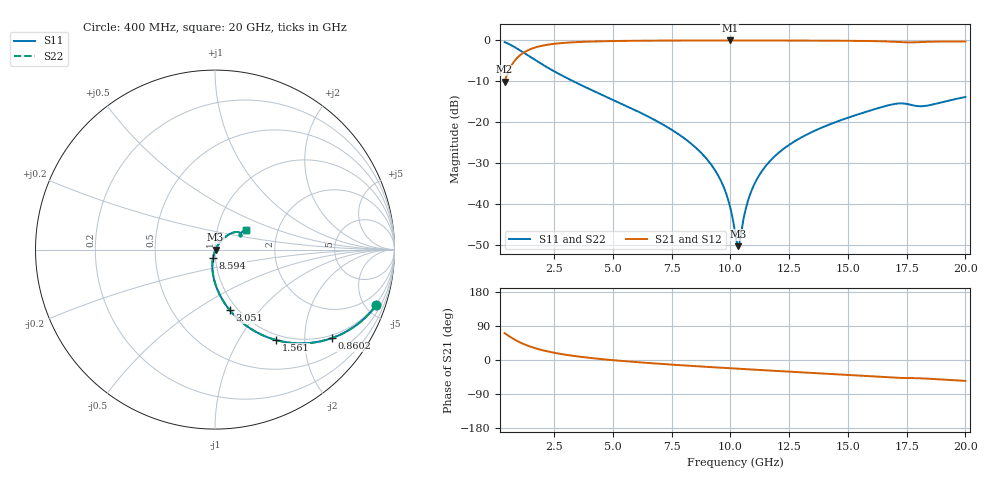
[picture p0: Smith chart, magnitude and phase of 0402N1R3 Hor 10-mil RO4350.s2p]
# GHz S MA R 50
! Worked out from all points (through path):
!   1960 points, 400 MHz to 20 GHz, reference 50 ohm
!   highest |S21| = -0.03 dB at 9.975 GHz (marker M1); lowest = -10.1 dB at 400 MHz (marker M2)
!   group delay of S21, straight-line fit = 12.9 ps
!   lowest |S11| = -50.3 dB at 10.34 GHz (marker M3), VSWR 1.01, Z = 50.3 - j0.116 ohm
!   |S11| at or under -10 dB: 3.318 GHz to end of sweep
!   |S22| runs from -50.3 to -0.4 dB; largest |S21 - S12| = 0
!   S11 on the Smith chart (normalised r, x): 400 MHz: 0.91, -5.82; 860.2 MHz: 0.91, -2.69; 1.561 GHz: 0.91, -1.46; 3.051 GHz: 0.92, -0.70; 8.594 GHz: 0.97, -0.09; 20 GHz: 1.38, +0.31
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0.4  0.9502 -19.0  0.3115 70.9  0.3115 70.9  0.9502 -19.0
0.8602348  0.8157 -37.2  0.5779 52.7  0.5779 52.7  0.8157 -37.2
1.560592  0.6081 -56.0  0.7928 33.9  0.7928 33.9  0.6081 -56.0
2.210924  0.4677 -66.9  0.8826 22.9  0.8826 22.9  0.4677 -66.9
3.051353  0.3456 -76.4  0.9367 13.4  0.9367 13.4  0.3456 -76.4
3.671669  0.2822 -81.5  0.9575 8.1  0.9575 8.1  0.2822 -81.5
6.943338  0.1005 -98.4  0.9922 -9.8  0.9922 -9.8  0.1005 -98.4
8.594181  0.04703 -103.2  0.9958 -16.5  0.9958 -16.5  0.04703 -103.2
9.444615  0.02335 -102.7  0.9964 -19.8  0.9964 -19.8  0.02335 -102.7
9.744768  0.01546 -99.9  0.9965 -20.9  0.9965 -20.9  0.01546 -99.9
9.974885  0.009648 -93.7  0.9965 -21.7  0.9965 -21.7  0.009648 -93.7
10.205  0.004449 -69.6  0.9965 -22.6  0.9965 -22.6  0.004449 -69.6
10.33507  0.003059 -22.1  0.9965 -23.0  0.9965 -23.0  0.003059 -22.1
10.4051  0.003573 7.4  0.9965 -23.3  0.9965 -23.3  0.003573 7.4
10.61521  0.007754 42.2  0.9964 -24.1  0.9964 -24.1  0.007754 42.2
10.7853  0.01176 49.8  0.9963 -24.7  0.9963 -24.7  0.01176 49.8
11.30556  0.0243 55.7  0.996 -26.5  0.996 -26.5  0.0243 55.7
12.17601  0.04511 55.9  0.995 -29.6  0.995 -29.6  0.04511 55.9
13.46667  0.07572 52.8  0.9925 -34.1  0.9925 -34.1  0.07572 52.8
16.73834  0.1613 37.3  0.9674 -45.9  0.9674 -45.9  0.1613 37.3
18.24911  0.1575 30.1  0.9566 -48.7  0.9566 -48.7  0.1575 30.1
20  0.2034 31.9  0.9679 -55.1  0.9679 -55.1  0.2034 31.9
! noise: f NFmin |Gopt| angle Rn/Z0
0.4  0.001319  0.8147  5.044  0.001484
2.571  0.005092  0.6816  7.72  0.003083
4.752  0.008087  0.6382  11.91  0.004173
6.933  0.01078  0.6118  16.27  0.005058
9.104  0.01334  0.5947  20.6  0.005863
11.29  0.01597  0.5861  24.91  0.006742
13.47  0.01931  0.5935  29.19  0.008197
15.64  0.02796  0.6634  33.76  0.01462
17.82  0.07029  0.8337  38.8  0.07949
20  0.03707  0.6803  42.51  0.01959
